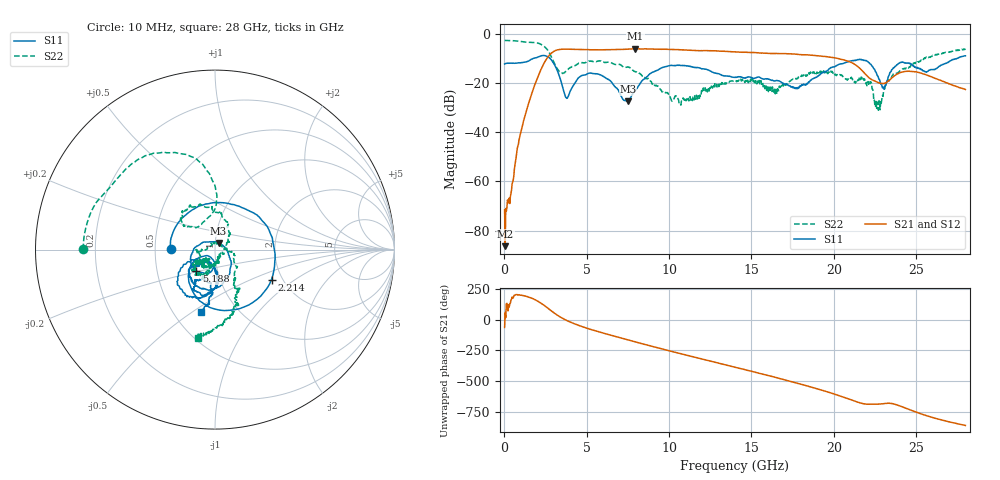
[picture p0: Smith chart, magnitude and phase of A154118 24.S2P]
!  2-Port S-parameters saved by WinCal
! VAR MeasName=S-Parameters (CALIBRATED_DATA) read from VNA (N5230A)
! VAR MeasDate=2015-9-10 14:36:10
! VAR NAME=A154118 24
! VAR FILENAME=A154118 24.S2P
! VAR DATE=2015-9-10 14:36:10
! VAR PHYS_PORTS=1,2
# Hz S DB R 50
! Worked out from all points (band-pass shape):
!   801 points, 10 MHz to 28 GHz, reference 50 ohm
!   highest |S21| = -6.07 dB at 7.952 GHz (marker M1); lowest = -86.4 dB at 44.99 MHz (marker M2)
!   |S21| within 3 dB of the highest: 2.676 GHz to 19.26 GHz (16.58 GHz wide, 151 % of centre)
!   lowest |S11| = -27.4 dB at 7.497 GHz (marker M3), VSWR 1.09, Z = 51.9 + j3.9 ohm
!   |S11| at or under -10 dB: start of sweep to 1.747 GHz; 2.771 GHz to 27.48 GHz (24.71 GHz wide, 163 % of centre)
!   |S22| runs from -31.1 to -2.7 dB; largest |S21 - S12| = 0.008
!   S11 on the Smith chart (normalised r, x): 10 MHz: 0.61, +0.00; 2.214 GHz: 1.76, -0.67; 5.188 GHz: 0.79, -0.20; 28 GHz: 0.68, -0.54
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1e7  -12.25 179.4  -71.57 -64.0  -69.30 -92.5  -2.67 179.9
4.49875e7  -12.15 177.2  -86.38 57.5  -86.97 141.8  -2.69 178.9
3.948625e8  -11.92 148.4  -64.92 157.5  -65.74 162.2  -2.73 170.3
1.094612e9  -11.67 88.9  -37.21 -164.3  -37.20 -163.9  -3.20 153.1
2.214212e9  -8.96 -27.9  -14.56 133.7  -14.54 134.2  -4.24 117.8
2.913962e9  -11.23 -114.7  -7.50 63.8  -7.47 63.8  -10.25 88.1
3.753662e9  -26.02 -132.0  -6.18 -5.5  -6.16 -5.4  -15.19 134.3
4.698325e9  -16.93 -109.9  -6.40 -56.2  -6.35 -56.2  -11.68 137.8
5.18815e9  -15.92 -130.8  -6.43 -78.1  -6.38 -78.1  -11.11 130.1
7.497325e9  -27.43 61.9  -6.20 -164.2  -6.16 -164.4  -13.40 81.1
7.952162e9  -22.93 -8.7  -6.07 178.8  -6.03 178.5  -15.50 68.7
9.351662e9  -14.60 -75.3  -6.30 129.1  -6.23 128.9  -21.60 32.1
1.068119e10  -12.87 -113.2  -6.48 83.5  -6.41 82.9  -28.54 -37.6
1.4005e10  -17.73 -138.4  -7.33 -27.0  -7.30 -27.4  -19.18 -119.0
1.631418e10  -19.00 -133.8  -7.98 -103.8  -7.95 -104.2  -22.25 -120.0
1.869332e10  -18.38 -86.7  -8.67 169.6  -8.70 169.2  -15.28 -112.8
2.023278e10  -12.64 -93.8  -9.99 106.7  -9.86 106.2  -16.77 -143.8
2.173724e10  -10.54 -126.6  -15.01 38.8  -15.01 37.3  -18.30 -142.4
2.26819e10  -17.12 -156.0  -19.79 33.3  -19.66 32.3  -27.99 103.1
2.334666e10  -17.04 -84.8  -19.06 41.1  -18.97 39.9  -18.67 -16.4
2.488611e10  -13.33 -119.6  -15.35 -25.0  -15.37 -25.9  -11.71 -61.0
2.8e10  -8.90 -103.0  -22.64 -139.6  -22.56 -140.6  -6.02 -101.0
